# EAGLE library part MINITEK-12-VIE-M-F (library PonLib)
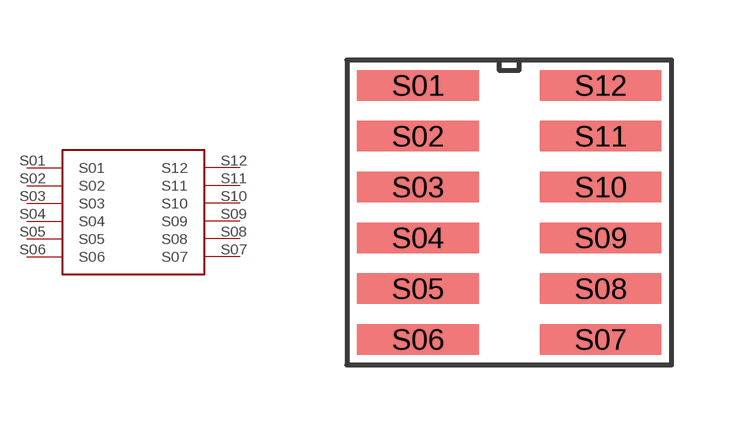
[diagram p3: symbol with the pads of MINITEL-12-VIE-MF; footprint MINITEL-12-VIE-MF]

Designator prefix -

## MINITEK-12-VIE-M-F  [MINITEL-12-VIE-MF]
S01  S01
S02  S02
S03  S03
S04  S04
S05  S05
S06  S06
S07  S07
S08  S08
S09  S09
S10  S10
S11  S11
S12  S12

## Footprint MINITEL-12-VIE-MF (pad centres in mm)
smd 3.048 x 0.762: S01 -2.286,3.175; S02 -2.286,1.905; S03 -2.286,0.635; S04 -2.286,-0.635; S05 -2.286,-1.905; S06 -2.286,-3.175; S07 2.286,-3.175; S08 2.286,-1.905; S09 2.286,-0.635; S10 2.286,0.635; S11 2.286,1.905; S12 2.286,3.175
